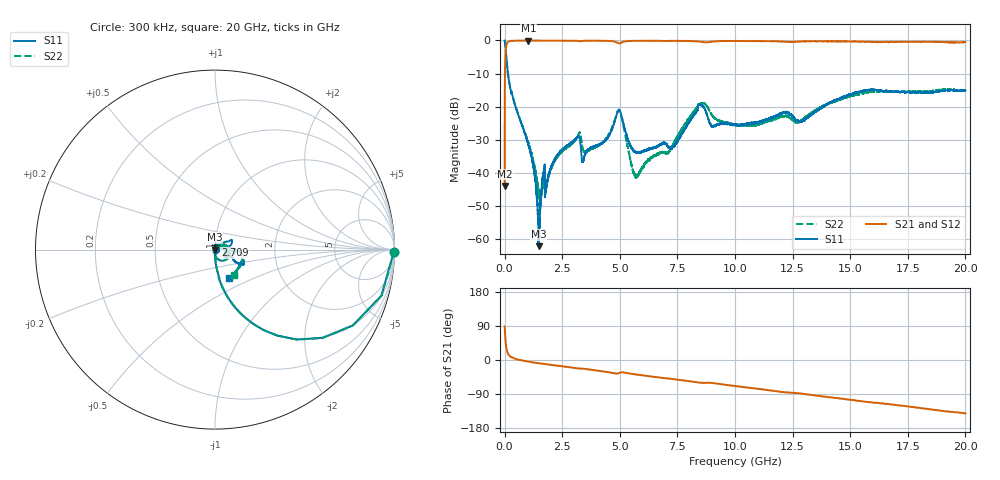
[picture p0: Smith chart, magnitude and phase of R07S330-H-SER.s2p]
!{R07S330}
!Johanson Technology Inc.
!www.johansontechnology.com
!Test Board Conditions:
!Substrate Type  RO4350B
!Substrate Thickness  10 mil
!Substrate Dk  3.66
!TL Type: GCPW
!TL Trace Width  21 mil
!TL Gap  20 mil
!Electrode orientation  Horizontal
!DUT TOPOLOGY	SERIES
!Mounting Pad LxW  16x21 mil
! Created Sat Feb  6 11:55:02 2021
# hz S ma R 50
! 2 Port Network Data from SP1.SP block
! freq  magS11  angS11  magS21  angS21  magS12  angS12  magS22  angS22
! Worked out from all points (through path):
!   20001 points, 300 kHz to 20 GHz, reference 50 ohm
!   highest |S21| = -0.03 dB at 1.034 GHz (marker M1); lowest = -44.0 dB at 300 kHz (marker M2)
!   group delay of S21, straight-line fit = 20.1 ps
!   lowest |S11| = -62.2 dB at 1.488 GHz (marker M3), VSWR 1.00, Z = 49.9 + j0.0293 ohm
!   |S11| at or under -10 dB: 144.1 MHz to end of sweep
!   |S22| runs from -48.7 to 0.0 dB; largest |S21 - S12| = 0.012
!   S11 on the Smith chart (normalised r, x): 300 kHz: open; 2.709 GHz: 1.00, +0.05; 20 GHz: 1.11, -0.36
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300000  0.9963 -0.7  0.006313 88.5  0.006144 89.3  0.9992 -0.8
1.013e8  0.4283 -65.3  0.902 24.8  0.903 24.7  0.4295 -65.1
1.333e8  0.3388 -71.1  0.9401 18.9  0.9404 18.9  0.3388 -70.9
1.0343e9  0.02619 -92.1  0.997 -4.5  0.996 -4.4  0.02822 -88.5
1.2613e9  0.01166 -96.2  0.9957 -6.6  0.9955 -6.6  0.01421 -83.4
1.4883e9  0.0007729 157.7  0.9951 -8.5  0.9956 -8.6  0.004988 -40.7
1.6493e9  0.008141 97.0  0.9955 -9.9  0.9951 -9.9  0.006338 31.9
2.7093e9  0.02568 85.0  0.9941 -18.3  0.9939 -18.2  0.02426 55.3
3.1793e9  0.03486 71.6  0.9857 -22.2  0.9856 -22.2  0.03582 41.5
3.3343e9  0.01883 44.0  0.9755 -22.3  0.9759 -22.3  0.03123 5.3
3.5063e9  0.01941 89.6  0.99 -23.7  0.9903 -23.6  0.02074 24.1
4.1933e9  0.0273 76.5  0.9885 -29.4  0.9896 -29.4  0.02754 33.8
4.9613e9  0.08794 -22.6  0.9064 -34.5  0.906 -34.5  0.08932 -22.7
5.6723e9  0.02057 -65.8  0.987 -38.0  0.9867 -37.9  0.009262 -169.0
6.6673e9  0.02529 -17.9  0.9867 -45.8  0.9871 -45.9  0.01898 75.7
7.3213e9  0.02477 14.3  0.9853 -50.5  0.9848 -50.5  0.02699 28.7
8.4893e9  0.1055 27.6  0.9578 -59.8  0.9577 -59.8  0.1096 4.3
9.0093e9  0.0497 31.0  0.9592 -60.6  0.9589 -60.7  0.07285 -22.8
1.00003e10  0.0533 28.3  0.981 -68.7  0.9825 -68.7  0.05226 6.9
1.33343e10  0.07586 -17.3  0.972 -92.3  0.9731 -92.4  0.08134 -5.5
1.66673e10  0.1671 -22.3  0.9394 -116.2  0.9456 -116.6  0.1681 -43.2
2e10  0.176 -63.0  0.9445 -140.8  0.9364 -140.7  0.1745 -53.8
